TYPE STR_HEATER_LINE :
STRUCT
	//INPUT
	Input_PV	AT%I*:	REAL	;
	Input_Temp_Hi_Alarm	AT%I*:	UINT	;
	Input_Working_Output	AT%I*:	REAL	;
	Input_Working_SP	AT%I*:	REAL	;
	Input_Inhibit_state	AT%I*:	BOOL	;
	Input_TC_Error	AT%I*:	BOOL	;
	Input_Auto_Manual	AT%I*:	BOOL	;
	Input_SBrkAlarm_EN	AT%I*:	USINT	;
	Input_Temp_Hi_Alarm_Inhibit	AT%I*:	USINT	;
	Input_Inhibit_Buffer	AT%I*:	REAL	;
	Input_RateUp	AT%I*:	REAL	;
	Input_RateDown	AT%I*:	REAL	;
	Input_AutotuneActivate	AT%I*:	USINT	;
	Input_Autotune_Status	AT%I*:	USINT	;
	Input_PID_P	AT%I*:	REAL	;
	Input_PID_I	AT%I*:	REAL	;
	Input_PID_D	AT%I*:	REAL	;
				
				
	//OUTPUT			
	Output_HEATER_SP	AT%Q*:	REAL	;
	Output_Clear_Alarms	AT%Q*:	UINT	;
	Output_Forced_MV	AT%Q*:	REAL	;
	Output_HEATER_Auto_Manual	AT%Q*:	BOOL 	;
	Output_HEATER_Inhibit	AT%Q*:	BOOL	;
	Output_HEATER_SBrkAlarm_EN	AT%Q*:	USINT	;
	Output_HEATER_Temp_Hi_Alarm_Inhibit	AT%Q*:	USINT	;
	Output_Inhibit_Buffer	AT%Q*:	REAL	;
	Output_HEATER_RateUp	AT%Q*:	REAL	;
	Output_HEATER_RateDown	AT%Q*:	REAL	;
	Output_HEATER_AutotuneActivate	AT%Q*:	USINT	;
	Output_HEATER_PID_P	AT%Q*:	REAL	;
	Output_HEATER_PID_I	AT%Q*:	REAL	;
	Output_HEATER_PID_D	AT%Q*:	REAL	;


END_STRUCT
END_TYPE
